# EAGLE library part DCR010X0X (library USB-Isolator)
DC/DC Converter DC010505 RS NR 5412.5189.00
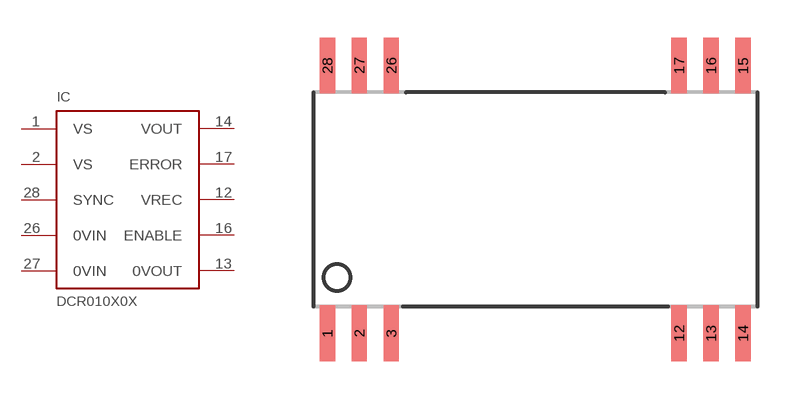
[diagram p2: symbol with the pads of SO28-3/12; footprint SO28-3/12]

Designator prefix IC

## DCR010X0X  [SO28-3/12]
1  VS
2  VS
12  VREC
13  0VOUT
14  VOUT
16  ENABLE
17  ERROR
26  0VIN
27  0VIN
28  SYNC

## Footprint SO28-3/12 (pad centres in mm)
Small Outline Package
smd 0.61 x 2.21: 1 -8.255,-5.315; 2 -6.985,-5.315; 3 -5.715,-5.315; 12 5.715,-5.315; 13 6.985,-5.315; 14 8.255,-5.315; 15 8.255,5.315; 16 6.985,5.315; 17 5.715,5.315; 26 -5.715,5.315; 27 -6.985,5.315; 28 -8.255,5.315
